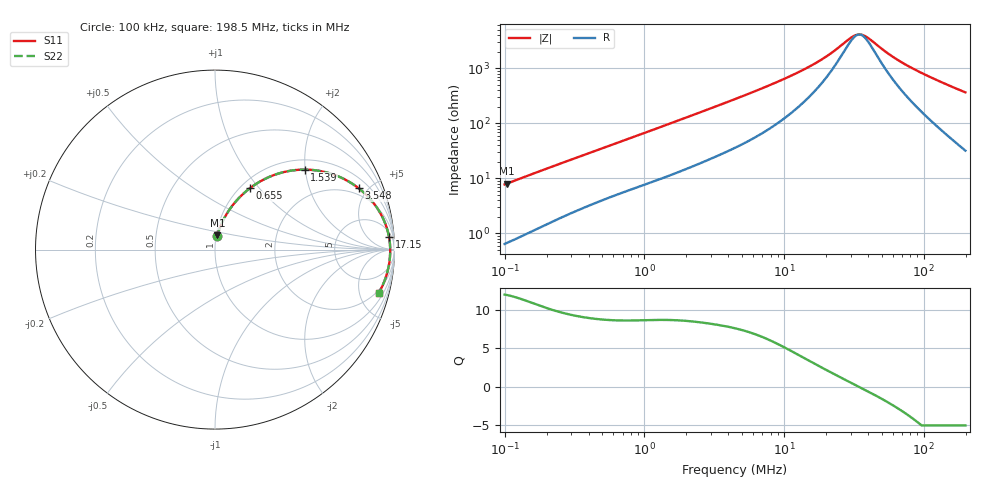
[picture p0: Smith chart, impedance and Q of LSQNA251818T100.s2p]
! LSQNA251818T100  S-PARAMETER MODEL  ( General Type )
! Model Generated by TAIYO YUDEN Corporation (http://www.ty-top.com)
! Version 2.0
! TAIYO YUDEN Control No. 100810NF25SB-FKC
! Copyright(c) 2007 TAIYO YUDEN CO.,LTD. All Rights Reserved.
! Product Description (link to TY-COMPAS)
! https://ds.yuden.co.jp/TYCOMPAS/or/detail?pn=LSQNA251818T100K&u=M
! Products Name : Inductors
! Characteristics :
!  Inductance : 10 uH , SRF(min) : 30 MHz , DC Resistance(max) : 0.325 Ohm
!  Rated Current : Saturation :250 mA , Temp Rise : 820 mA (40 degC)
!  Case Size : 2.5 x 1.8 / 0.098 x 0.071 [mm/inch] , Thickness : 1.8 / 0.071 [mm/inch]
!  (Conditions: Temperature = 25 degC , DC Bias Current/Voltage = 0A / 0V)
! External Node Assignments :
!  1  o---GGG---o  2
! GND o---------o GND
! Frequency Range : 0.1MHz  -  198.534594MHz  [ 402 STEP ]
# MHz S RI R 50
! Freq[MHz].  S11 Real  S11 Imag  S21 Real  S21 Imag  S12 Real  S12 Imag  S22 Real  S22 Imag
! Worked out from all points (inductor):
!   401 points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, 100 kHz to 198.5 MHz, reference 50 ohm
!   read as one part in series: L = 12.2 uH near 103.9 kHz
!   highest Q = 11.9 at 103.9 kHz (marker M1), where L = 12.3 uH
!   self-resonance near 34.51 MHz
!   S11 on the Smith chart (normalised r, x): 100 kHz: 1.01, +0.15; 655 kHz: 1.10, +0.90; 1.539 MHz: 1.23, +1.98; 3.548 MHz: 1.55, +4.38; 17.15 MHz: 9, +24; 198.5 MHz: 1.64, -7.26
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0.1  0.0122 0.0758  0.9878 -0.0758  0.9878 -0.0758  0.0122 0.0758
0.10387  0.0129 0.0786  0.9871 -0.0786  0.9871 -0.0786  0.0129 0.0786
0.194339  0.0339 0.1388  0.9661 -0.1388  0.9661 -0.1388  0.0339 0.1388
0.356769  0.0843 0.2281  0.9157 -0.2281  0.9157 -0.2281  0.0843 0.2281
0.65496  0.1953 0.3426  0.8047 -0.3426  0.8047 -0.3426  0.1953 0.3426
1.272844  0.4199 0.4393  0.5801 -0.4393  0.5801 -0.4393  0.4199 0.4393
1.538938  0.4991 0.4457  0.5009 -0.4457  0.5009 -0.4457  0.4991 0.4457
2.249639  0.654 0.4203  0.346 -0.4203  0.346 -0.4203  0.654 0.4203
3.547995  0.8012 0.3412  0.1988 -0.3412  0.1988 -0.3412  0.8012 0.3412
4.541117  0.8575 0.2897  0.1425 -0.2897  0.1425 -0.2897  0.8575 0.2897
9.16669  0.9445 0.1553  0.0555 -0.1553  0.0555 -0.1553  0.9445 0.1553
15.89665  0.968 0.0787  0.032 -0.0787  0.032 -0.0787  0.968 0.0787
17.15079  0.9697 0.0699  0.0303 -0.0699  0.0303 -0.0699  0.9697 0.0699
21.95147  0.9735 0.0434  0.0265 -0.0434  0.0265 -0.0434  0.9735 0.0434
30.3125  0.9759 0.0121  0.0241 -0.0121  0.0241 -0.0121  0.9759 0.0121
33.96951  0.9762 0.00146  0.0238 -0.00146  0.0238 -0.00146  0.9762 0.00146
36.64946  0.9763 -0.00563  0.0237 0.00563  0.0237 0.00563  0.9763 -0.00563
39.54085  0.9762 -0.0128  0.0238 0.0128  0.0238 0.0128  0.9762 -0.0128
56.71438  0.9742 -0.0482  0.0258 0.0482  0.0258 0.0482  0.9742 -0.0482
71.22432  0.9711 -0.0734  0.0289 0.0734  0.0289 0.0734  0.9711 -0.0734
94.68848  0.9641 -0.1098  0.0359 0.1098  0.0359 0.1098  0.9641 -0.1098
198.5346  0.9116 -0.2434  0.0884 0.2434  0.0884 0.2434  0.9116 -0.2434
